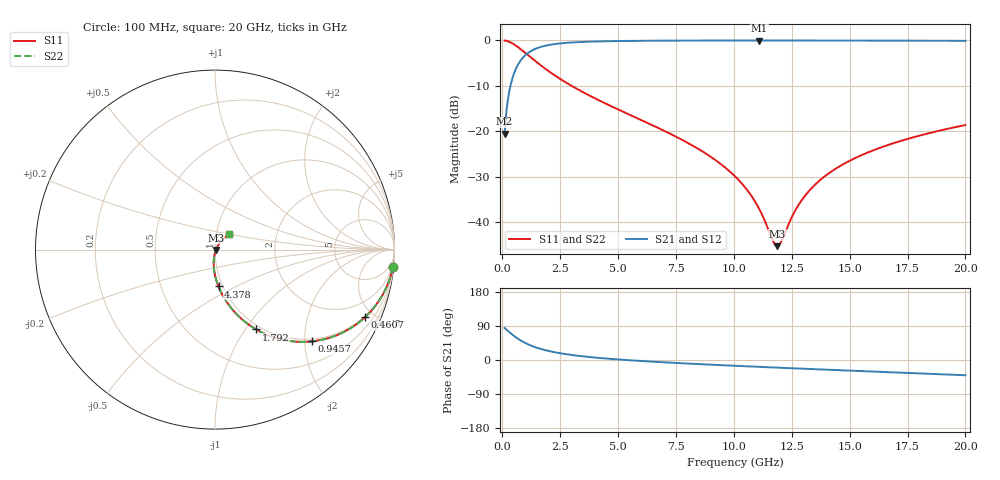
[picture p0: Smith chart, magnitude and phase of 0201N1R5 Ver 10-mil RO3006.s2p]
# GHz S MA R 50
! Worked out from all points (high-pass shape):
!   1601 points, 100 MHz to 20 GHz, reference 50 ohm
!   highest |S21| = -0.05 dB at 11.11 GHz (marker M1); lowest = -20.5 dB at 100 MHz (marker M2)
!   |S21| within 3 dB of the highest: 1.047 GHz to end of sweep
!   lowest |S11| = -45.3 dB at 11.88 GHz (marker M3), VSWR 1.01, Z = 50.5 - j0.189 ohm
!   |S11| at or under -10 dB: 2.986 GHz to end of sweep
!   |S22| runs from -45.3 to 0.0 dB; largest |S21 - S12| = 0
!   S11 on the Smith chart (normalised r, x): 100 MHz: 1, -21; 460.7 MHz: 0.94, -4.46; 945.8 MHz: 0.94, -2.16; 1.792 GHz: 0.95, -1.12; 4.378 GHz: 0.95, -0.41; 20 GHz: 1.16, +0.20
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0.1  0.9956 -5.6  0.09387 84.4  0.09387 84.4  0.9956 -5.6
0.2865625  0.9652 -15.6  0.2609 74.3  0.2609 74.3  0.9652 -15.6
0.4606875  0.9166 -24.3  0.3987 65.7  0.3987 65.7  0.9166 -24.3
0.672125  0.8433 -33.6  0.536 56.3  0.536 56.3  0.8433 -33.6
0.94575  0.7435 -43.4  0.6669 46.4  0.6669 46.4  0.7435 -43.4
1.34375  0.614 -54.2  0.7871 35.6  0.7871 35.6  0.614 -54.2
1.7915  0.5003 -62.7  0.8632 27.0  0.8632 27.0  0.5003 -62.7
2.475563  0.3793 -71.5  0.9222 18.1  0.9222 18.1  0.3793 -71.5
3.420812  0.2743 -79.2  0.9581 10.1  0.9581 10.1  0.2743 -79.2
4.3785  0.2063 -84.5  0.9746 4.4  0.9746 4.4  0.2063 -84.5
6.741625  0.1083 -93.0  0.9896 -5.3  0.9896 -5.3  0.1083 -93.0
8.719188  0.05828 -96.8  0.9933 -11.5  0.9933 -11.5  0.05828 -96.8
10.05  0.03189 -96.1  0.9942 -15.3  0.9942 -15.3  0.03189 -96.1
11.10719  0.01379 -85.6  0.9943 -18.1  0.9943 -18.1  0.01379 -85.6
11.69175  0.006189 -48.8  0.9943 -19.7  0.9943 -19.7  0.006189 -48.8
11.87831  0.00544 -20.1  0.9943 -20.2  0.9943 -20.2  0.00544 -20.1
12.05244  0.006147 6.5  0.9942 -20.6  0.9942 -20.6  0.006147 6.5
12.7365  0.01462 45.1  0.994 -22.4  0.994 -22.4  0.01462 45.1
13.37081  0.02383 52.2  0.9937 -24.0  0.9937 -24.0  0.02383 52.2
14.7265  0.04339 54.8  0.9927 -27.4  0.9927 -27.4  0.04339 54.8
16.69162  0.07099 52.7  0.9908 -32.2  0.9908 -32.2  0.07099 52.7
20  0.117 46.4  0.9858 -40.2  0.9858 -40.2  0.117 46.4
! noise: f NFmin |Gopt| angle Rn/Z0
0.1  0.0009744  0.9578  0.7687  0.005206
2.301  0.005359  0.8261  4.404  0.00647
4.515  0.008286  0.7844  8.06  0.007857
6.729  0.01081  0.7577  11.72  0.008936
8.943  0.01311  0.7382  15.37  0.009851
11.14  0.01527  0.7232  18.96  0.01066
13.36  0.01735  0.7112  22.54  0.01139
15.57  0.01937  0.7015  26.08  0.01208
17.79  0.02134  0.6936  29.58  0.01272
20  0.02329  0.6873  33.03  0.01334
